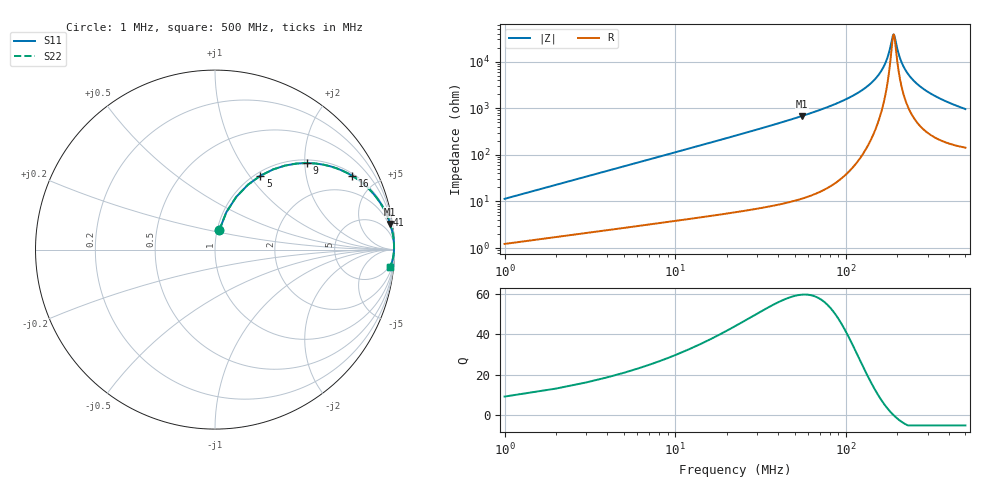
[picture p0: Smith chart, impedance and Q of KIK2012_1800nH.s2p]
!version-2
!date-01.2022
!Series
# MHz S RI R 50
!Freq ReS11 ImS11 ReS21 ImS21 ReS12 ImS12 ReS22 ImS22
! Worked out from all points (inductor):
!   500 points, 1 MHz to 500 MHz, reference 50 ohm
!   read as one part in series: L = 1.8 uH near 3 MHz
!   highest Q = 59.4 at 55 MHz (marker M1), where L = 1.96 uH
!   self-resonance near 190 MHz
!   S11 on the Smith chart (normalised r, x): 1 MHz: 1.02, +0.23; 5 MHz: 1.05, +1.13; 9 MHz: 1.07, +2.04; 16 MHz: 1.10, +3.64; 41 MHz: 1.17, +9.73; 500 MHz: 4, -19
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1  0.0243 0.109  0.9757 -0.109  0.9757 -0.109  0.0243 0.109
5  0.2531 0.4116  0.7469 -0.4116  0.7469 -0.4116  0.2531 0.4116
9  0.5099 0.4825  0.4901 -0.4825  0.4901 -0.4825  0.5099 0.4825
16  0.7628 0.4122  0.2372 -0.4122  0.2372 -0.4122  0.7628 0.4122
25  0.8871 0.3059  0.1129 -0.3059  0.1129 -0.3059  0.8871 0.3059
41  0.9562 0.1958  0.0438 -0.1958  0.0438 -0.1958  0.9562 0.1958
55  0.9765 0.1434  0.0235 -0.1434  0.0235 -0.1434  0.9765 0.1434
85  0.9915 0.0823  0.00848 -0.0823  0.00848 -0.0823  0.9915 0.0823
139  0.9974 0.0295  0.00264 -0.0295  0.00264 -0.0295  0.9974 0.0295
168  0.9977 0.0115  0.00231 -0.0115  0.00231 -0.0115  0.9977 0.0115
176  0.9976 0.00716  0.00237 -0.00716  0.00237 -0.00716  0.9976 0.00716
187  0.9975 0.00155  0.00254 -0.00155  0.00254 -0.00155  0.9975 0.00155
190  0.9974 8.39e-05  0.0026 -8.39e-05  0.0026 -8.39e-05  0.9974 8.39e-05
193  0.9973 -0.00136  0.00266 0.00136  0.00266 0.00136  0.9973 -0.00136
204  0.9971 -0.00648  0.00294 0.00648  0.00294 0.00648  0.9971 -0.00648
214  0.9967 -0.0109  0.00326 0.0109  0.00326 0.0109  0.9967 -0.0109
230  0.9961 -0.0176  0.00386 0.0176  0.00386 0.0176  0.9961 -0.0176
251  0.9952 -0.0258  0.0048 0.0258  0.0048 0.0258  0.9952 -0.0258
286  0.9933 -0.0383  0.00673 0.0383  0.00673 0.0383  0.9933 -0.0383
334  0.99 -0.0539  0.00995 0.0539  0.00995 0.0539  0.99 -0.0539
417  0.9831 -0.0776  0.0169 0.0776  0.0169 0.0776  0.9831 -0.0776
500  0.9748 -0.0988  0.0252 0.0988  0.0252 0.0988  0.9748 -0.0988
